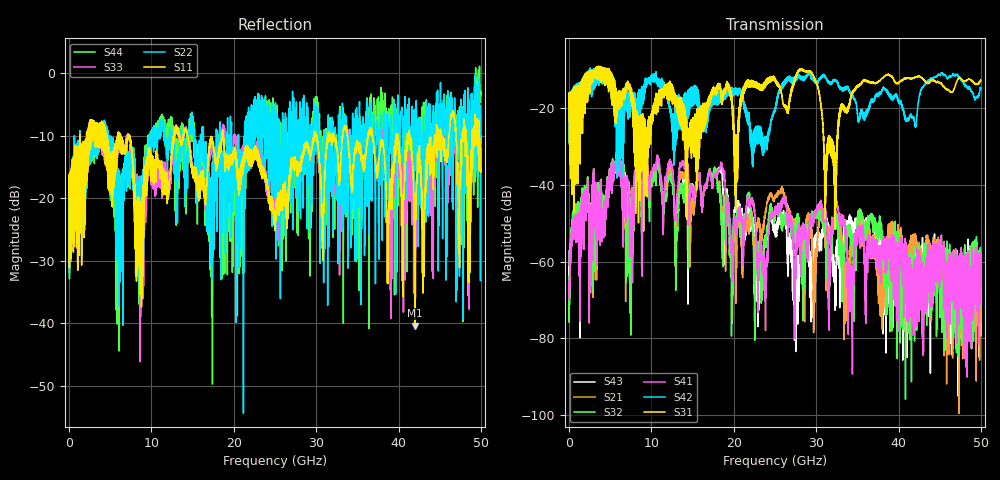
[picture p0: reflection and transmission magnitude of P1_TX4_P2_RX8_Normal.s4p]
!Keysight Technologies,N5225B,MY57041031,A.13.20.10
!Date: Friday, May 31, 2019 11:40:25
!Correction: S11(Full 4 Port(1,2,3,4))
!S12(Full 4 Port(1,2,3,4))
!S13(Full 4 Port(1,2,3,4))
!S14(Full 4 Port(1,2,3,4))
!S21(Full 4 Port(1,2,3,4))
!S22(Full 4 Port(1,2,3,4))
!S23(Full 4 Port(1,2,3,4))
!S24(Full 4 Port(1,2,3,4))
!S31(Full 4 Port(1,2,3,4))
!S32(Full 4 Port(1,2,3,4))
!S33(Full 4 Port(1,2,3,4))
!S34(Full 4 Port(1,2,3,4))
!S41(Full 4 Port(1,2,3,4))
!S42(Full 4 Port(1,2,3,4))
!S43(Full 4 Port(1,2,3,4))
!S44(Full 4 Port(1,2,3,4))
!S4P File: Measurements: <S11,S12,S13,S14>,
!<S21,S22,S23,S24>,
!<S31,S32,S33,S34>,
!<S41,S42,S43,S44>:
# Hz S  dB  R 50.0
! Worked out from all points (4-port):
!   5000 points, 10 MHz to 50 GHz, reference 50 ohm
!   strongest paths, dB at 10 MHz, 12.51 GHz, 25.01 GHz, 37.51 GHz, 50 GHz:
!     S31: -19.6, -17.6, -12.9, -13.0, -12.6
!     S42: -19.6, -21.7, -19.9, -16.4, -15.0
!     S41: -67.3, -36.2, -45.8, -57.6, -58.8
!     S32: -66.5, -39.4, -49.4, -54.9, -69.1
!     S21: -64.8, -38.0, -43.2, -60.5, -64.9
!     S43: -57.2, -37.8, -50.8, -55.6, -79.4
!   lowest |S11| = -40.3 dB at 42 GHz (marker M1), VSWR 1.02, Z = 49.2 + j0.588 ohm
!   |S11| at or under -10 dB: 7.336 GHz to 12.7 GHz (5.362 GHz wide, 53.5 % of centre); 14.41 GHz to 18.57 GHz (4.156 GHz wide, 25.2 % of centre); 18.74 GHz to 29.76 GHz (11.02 GHz wide, 45.4 % of centre)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
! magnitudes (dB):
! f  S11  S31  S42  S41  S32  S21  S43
! 10 MHz  -19.6  -19.6  -19.6  -67.3  -66.5  -64.8  -57.2
! 10.73 GHz  -13.4  -17.6  -13.4  -32.7  -34.3  -33.2  -33.7
! 18.33 GHz  -11.6  -13.7  -17.9  -35.7  -42.4  -41.8  -36.3
! 23.03 GHz  -13.9  -15.0  -25.9  -63.5  -56.2  -51.0  -72.7
! 32.24 GHz  -10.4  -36.0  -12.5  -47.9  -50.8  -49.6  -61.5
! 42 GHz  -40.3  -12.0  -24.8  -70.9  -67.0  -53.8  -54.6
! 50 GHz  -12.1  -12.6  -15.0  -58.8  -69.1  -64.9  -79.4
